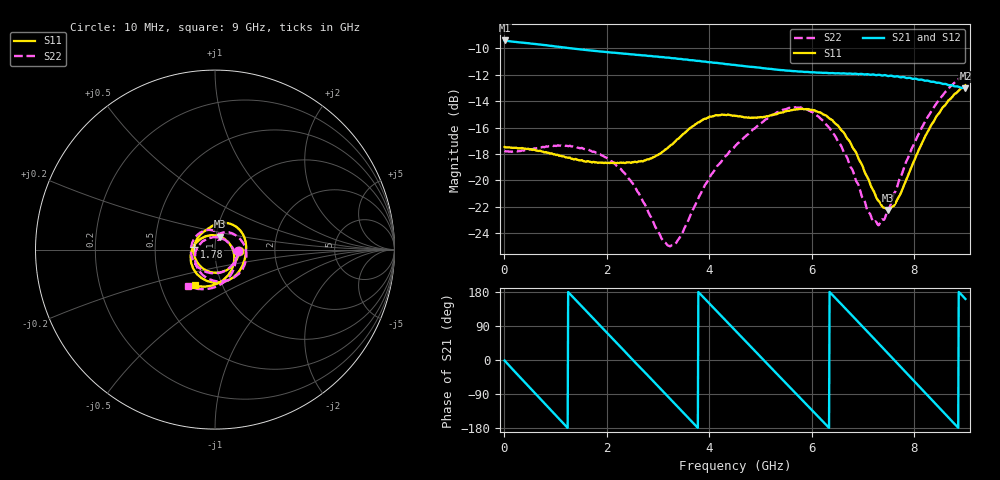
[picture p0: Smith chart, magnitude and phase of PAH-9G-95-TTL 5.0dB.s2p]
! MTS Systemtechnik GmbH
! S-Parameters
! Model: PAH-9G/95-TTL
! Attenuation Step: 5.0dB
#  HZ  S  DB  R  50.00
! Rohde & Schwarz Vector Network Analyzer
! Rohde-Schwarz,ZNB20-2Port,1334333062101652,3.45
! Created: UTC 1/26/2024, 7:18:37 AM
! freq[Hz]  db:S11  ang:S11  db:S21  ang:S21  db:S12  ang:S12  db:S22  ang:S22
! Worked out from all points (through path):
!   900 points, 10 MHz to 9 GHz, reference 50 ohm
!   highest |S21| = -9.41 dB at 10 MHz (marker M1); lowest = -13.0 dB at 9 GHz (marker M2)
!   group delay of S21, straight-line fit = 393 ps
!   lowest |S11| = -22.2 dB at 7.49 GHz (marker M3), VSWR 1.17, Z = 52.3 + j7.58 ohm
!   |S11| at or under -10 dB: start of sweep to end of sweep
!   |S22| runs from -25.0 to -12.0 dB; largest |S21 - S12| = 0.0094
!   S11 on the Smith chart (normalised r, x): 10 MHz: 1.31, -0.02; 1.78 GHz: 0.79, +0.03; 9 GHz: 0.74, -0.31
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1e7  -17.47 -2.4  -9.41 -1.4  -9.41 -1.5  -17.75 -2.9
3.8e8  -17.59 -48.7  -9.58 -55.7  -9.59 -55.6  -17.74 -57.2
6.8e8  -17.77 -85.2  -9.71 -99.0  -9.72 -98.9  -17.55 -99.6
1.12e9  -18.17 -132.8  -9.92 -162.1  -9.92 -161.9  -17.37 -154.4
1.51e9  -18.47 -167.3  -10.09 142.3  -10.10 142.5  -17.54 164.0
1.78e9  -18.63 172.2  -10.20 104.1  -10.21 104.2  -17.88 139.0
2.43e9  -18.63 131.2  -10.44 11.7  -10.45 12.4  -19.86 88.4
3.01e9  -18.05 104.3  -10.64 -70.1  -10.65 -70.0  -23.91 66.5
3.34e9  -17.04 88.5  -10.76 -117.1  -10.77 -116.5  -24.79 76.8
3.76e9  -15.69 63.4  -10.95 -176.4  -10.95 -175.9  -21.59 76.8
4.18e9  -15.07 35.2  -11.13 124.4  -11.13 124.8  -18.83 58.3
4.51e9  -15.11 13.7  -11.26 77.9  -11.27 78.3  -17.39 39.9
5.16e9  -15.14 -24.5  -11.55 -13.7  -11.56 -12.7  -15.25 -2.4
5.6e9  -14.69 -54.0  -11.71 -75.3  -11.72 -74.3  -14.52 -38.8
6.01e9  -14.68 -88.6  -11.81 -132.9  -11.83 -131.7  -14.82 -78.3
6.42e9  -15.51 -128.7  -11.88 169.6  -11.89 170.7  -16.44 -123.4
6.86e9  -17.83 -179.9  -11.92 107.2  -11.95 108.6  -19.96 177.6
7.21e9  -20.80 126.3  -11.98 57.6  -12.02 58.5  -23.16 108.3
7.49e9  -22.24 68.9  -12.10 17.5  -12.09 18.7  -22.15 43.6
7.51e9  -22.22 64.2  -12.10 14.8  -12.08 15.8  -22.07 39.7
8.23e9  -16.56 -53.3  -12.45 -89.0  -12.45 -87.4  -15.44 -60.4
9e9  -12.80 -119.1  -13.04 161.1  -13.08 162.8  -11.97 -126.6
